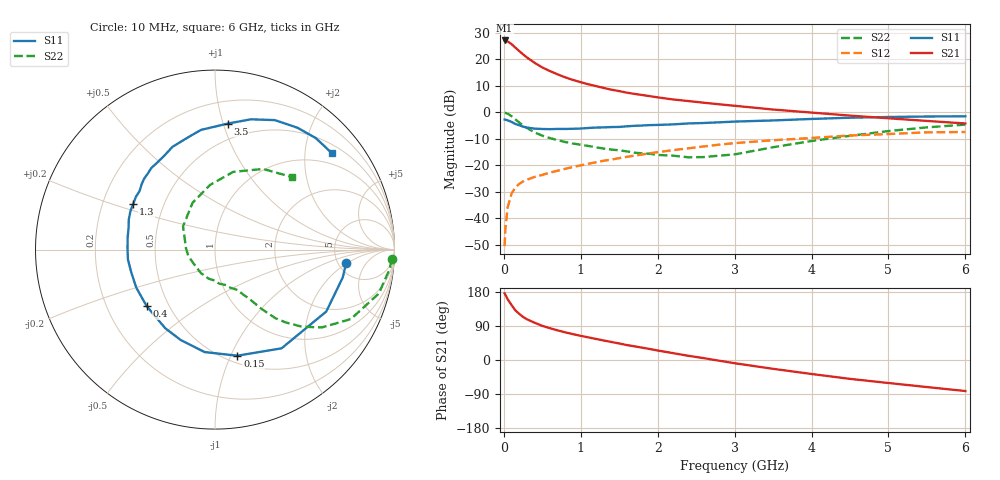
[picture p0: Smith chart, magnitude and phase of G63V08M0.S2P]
! SIEMENS Small Signal Semiconductors
! BFG193
! Si NPN RF Bipolar Junction Transistor in SOT223
! VCE = 3 V  IC = 8 mA
! Common Emitter S-Parameters:  August  1996
# GHz  S  MA  R  50
!  f  S11  S21  S12  S22
! GHz  MAG  ANG  MAG  ANG  MAG  ANG  MAG  ANG
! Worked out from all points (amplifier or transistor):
!   36 points, 10 MHz to 6 GHz, reference 50 ohm
!   highest |S21| = 27.1 dB at 10 MHz (marker M1)
!   |S21| within 3 dB of that: start of sweep to 161 MHz
!   unconditionally stable (mu >= 1): 942 MHz to 2.555 GHz
!   at 250 MHz: K = 0.47, MSG = 24.0 dB, |S12| = -26.1 dB
!   at 1.4 GHz: K = 1.08, MAG = 11.5 dB, |S12| = -17.8 dB
!   at 6 GHz: K = 0.88, MSG = 1.6 dB, |S12| = -7.4 dB
!   S11 on the Smith chart (normalised r, x): 10 MHz: 5.85, -1.95; 150 MHz: 0.57, -1.06; 400 MHz: 0.38, -0.31; 1.3 GHz: 0.33, +0.23; 3.5 GHz: 0.37, +1.04; 6 GHz: 0.70, +2.62
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0.01  0.734 -6.0  22.77 175.8  0.003 93.3  0.9858 -3.1
0.02  0.7286 -12.3  22.67 172.5  0.0066 81.5  0.98 -6.2
0.05  0.7095 -29.1  21.77 160.1  0.0162 76.1  0.9451 -15.0
0.1  0.6634 -56.0  19.45 145.1  0.0295 65.7  0.8499 -27.1
0.15  0.6041 -78.1  16.64 131.0  0.0385 57.4  0.7363 -36.1
0.2  0.5738 -95.8  14.4 121.8  0.0449 52.8  0.6467 -41.6
0.25  0.5389 -110.7  12.45 113.6  0.0498 49.4  0.5646 -45.9
0.3  0.5185 -122.3  10.88 107.5  0.0537 48.0  0.5075 -48.7
0.4  0.4942 -140.4  8.619 98.3  0.0607 46.3  0.42 -51.9
0.5  0.4871 -154.2  7.054 90.1  0.0664 45.5  0.3643 -53.8
0.6  0.4835 -164.8  6.014 83.9  0.0733 46.2  0.3278 -55.5
0.7  0.4883 -173.5  5.218 78.1  0.0795 46.5  0.2999 -57.6
0.9  0.4913 172.2  4.094 68.2  0.0936 46.3  0.259 -60.8
1.1  0.5088 160.7  3.389 59.6  0.1075 45.9  0.2328 -67.1
1.3  0.5217 150.9  2.89 51.4  0.1228 44.8  0.2075 -72.7
1.6  0.5475 138.3  2.358 39.4  0.1454 41.5  0.1841 -85.8
2.2  0.5948 118.3  1.754 18.1  0.1944 32.8  0.1528 -120.6
2.8  0.6502 101.6  1.422 -1.9  0.2465 21.6  0.153 -167.3
3.5  0.7058 84.2  1.134 -23.3  0.2985 5.8  0.2205 143.9
4.5  0.7947 65.2  0.871 -49.8  0.367 -14.1  0.3617 94.3
5.5  0.8374 47.9  0.691 -71.4  0.4214 -38.7  0.5227 59.3
6  0.8443 39.5  0.619 -81.9  0.4275 -52.8  0.5886 43.5
